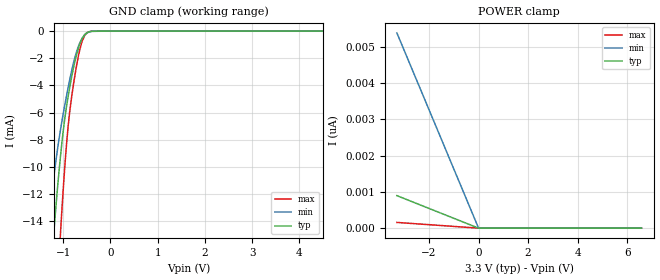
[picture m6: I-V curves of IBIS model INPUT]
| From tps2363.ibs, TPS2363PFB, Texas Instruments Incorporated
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|   INPUT MODEL
[Model]   INPUT
Model_type   Input
|   VALID FOR SCL, ONA, ONB, AUXENA, AUXENB
Vinl = 0.8V
Vinh = 2.0V
|   typ   min   max
C_comp   2.564pF   2.699pF   2.439pF
[Voltage Range]   3.300V   3.000V   3.600V
|Junction Temperature
[Temperature Range]   40.0   125.0   -40.0
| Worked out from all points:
|   GND clamp passes 1 mA (typ) near -0.66 V on its own axis
[GND Clamp]
|   Voltage   I(typ)   I(min)   I(max)
-3.3V     -183.6mA   -124.8mA   -259.9mA
-1.34V    -21.69mA   -15.01mA   -35.39mA
-1.191V   -14.45mA   -10.49mA   -23.67mA
-1.063V   -9.34mA    -7.337mA   -15.11mA
-1.053V   -9mA       -7.126mA   -14.52mA
-973.5mV  -6.59mA    -5.552mA   -10.27mA
-914.1mV  -5.174mA   -4.461mA   -7.659mA
-815.1mV  -3.245mA   -2.806mA   -4.658mA
-716.1mV  -1.706mA   -1.495mA   -2.493mA
-617.1mV  -662.1uA   -634.8uA   -929.3uA
-468.6mV  -66.1uA    -90.85uA   -71.68uA
6.58V     0A         0A         0A
[POWER Clamp]
|   Voltage   I(typ)   I(min)   I(max)
-3.3V     897.9pA    5.39nA     158.4pA
0V        0A         0A         0A
6.58V     0A         0A         0A
